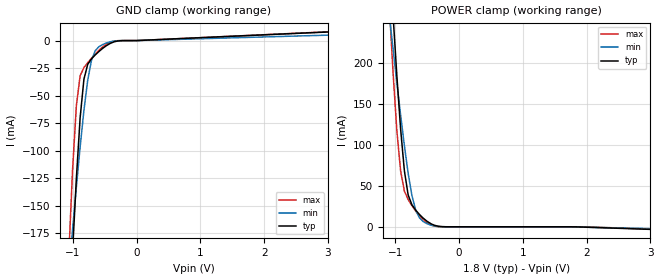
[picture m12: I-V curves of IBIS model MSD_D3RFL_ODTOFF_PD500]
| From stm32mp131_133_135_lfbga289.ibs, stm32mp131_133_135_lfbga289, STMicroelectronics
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[Model] MSD_D3RFL_ODTOFF_PD500
Model_type   Input
C_comp 2.366pF   2.308pF   2.512pF
Vinh = 1.440V
Vinl = 360.000mV
[Temperature Range]   25.000   125.000   -40.000
[Voltage Range]   1.800V   1.650V   1.950V
[GND Clamp Reference]   0.00V   0.00V   0.00V
[POWER Clamp Reference]   1.800V   1.650V   1.950V
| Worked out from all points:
|   GND clamp passes 1 mA (typ) near -0.34 V on its own axis
|   POWER clamp passes 1 mA (typ) near -0.35 V on its own axis
[GND Clamp]
-1.773V   -1.215A    -712.9mA   -1.314A
-1.064V   -264.1mA   -211.1mA   -194.1mA
-1.005V   -191.6mA   -171.4mA   -117.2mA
-945.5mV  -125mA     -133mA     -59.01mA
-886.4mV  -70mA      -96.59mA   -31.92mA
-827.3mV  -35.16mA   -63.52mA   -24.56mA
-768.2mV  -21.67mA   -36.21mA   -20.14mA
-709.1mV  -16.62mA   -17.94mA   -16.1mA
-650mV    -13.05mA   -9.189mA   -12.3mA
-531.8mV  -7.007mA   -3.566mA   -5.732mA
-236.4mV  -79.72uA   -39.83uA   -9.121uA
3.545V    9.219mA    5.818mA    9.435mA
[Power Clamp]
-1.745V   1.221A     726mA      1.304A
-1.095V   334mA      257.3mA    268.5mA
-1.036V   257mA      216.1mA    186.9mA
-977.3mV  184mA      175.6mA    117mA
-918.2mV  118.9mA    136.2mA    67.91mA
-859.1mV  68.16mA    98.81mA    43.59mA
-800mV    38.72mA    65.14mA    33.18mA
-740.9mV  26.77mA    38.03mA    25.67mA
-681.8mV  20.22mA    20.19mA    19.12mA
-563.6mV  10.47mA    6.377mA    8.639mA
-268.2mV  158uA      93.73uA    30.24uA
3.573V    -4.677mA   -3.227mA   -4.35mA
